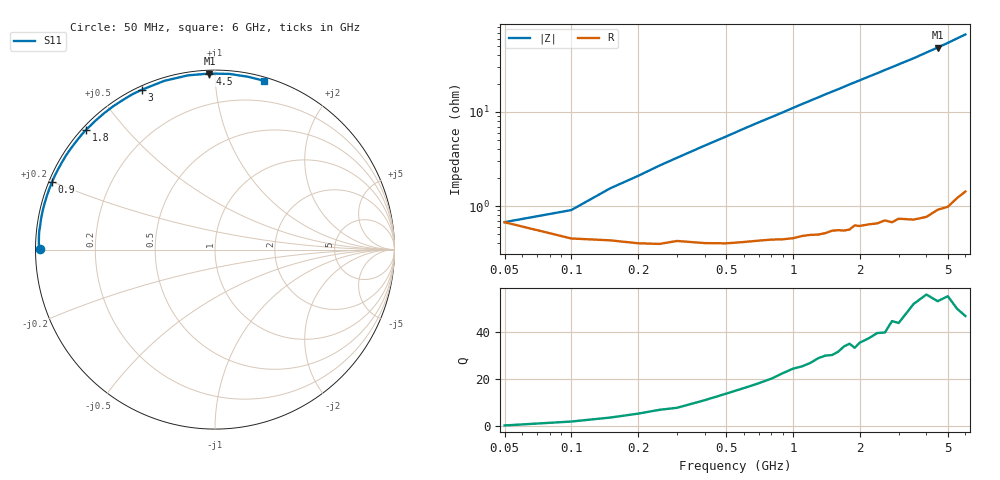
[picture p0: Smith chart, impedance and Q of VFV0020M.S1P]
! Infineon Technologies  Discrete & RF Semiconductors
! BBY 58-03
! Si Tuning Diode in SOD323
! VR =
! S-Parameters:  June  1999
# GHz  S  MA  R  50
!  f  S11
! GHz  MAG  ANG
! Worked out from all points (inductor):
!   34 points, 50 MHz to 6 GHz, reference 50 ohm
!   read as one part to ground: L = 1.63 nH near 150 MHz
!   highest Q = 55.2 at 4.5 GHz (marker M1), where L = 1.71 nH
!   S11 on the Smith chart (normalised r, x): 50 MHz: 0.01, +0.00; 900 MHz: 0.01, +0.20; 1.8 GHz: 0.01, +0.39; 3 GHz: 0.01, +0.64; 4.5 GHz: 0.02, +0.97; 6 GHz: 0.03, +1.33
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0.05  0.9735 179.9
0.1  0.9821 178.2
0.15  0.9829 176.6
0.2  0.9841 175.3
0.25  0.9843 173.9
0.4  0.9841 170.0
0.5  0.9843 167.5
0.6  0.9838 164.9
0.8  0.9831 160.0
0.9  0.9831 157.6
1  0.9828 155.1
1.1  0.982 152.7
1.3  0.9818 148.1
1.4  0.9814 145.8
1.6  0.9804 141.5
1.8  0.9807 137.1
2  0.9796 133.1
2.2  0.9794 129.1
2.4  0.9796 125.4
2.6  0.9788 121.6
2.8  0.9804 118.1
3  0.9794 114.6
3.5  0.9817 106.7
4  0.9825 98.8
4.5  0.9813 91.8
5  0.9821 85.3
5.5  0.9805 79.1
6  0.9797 73.7
